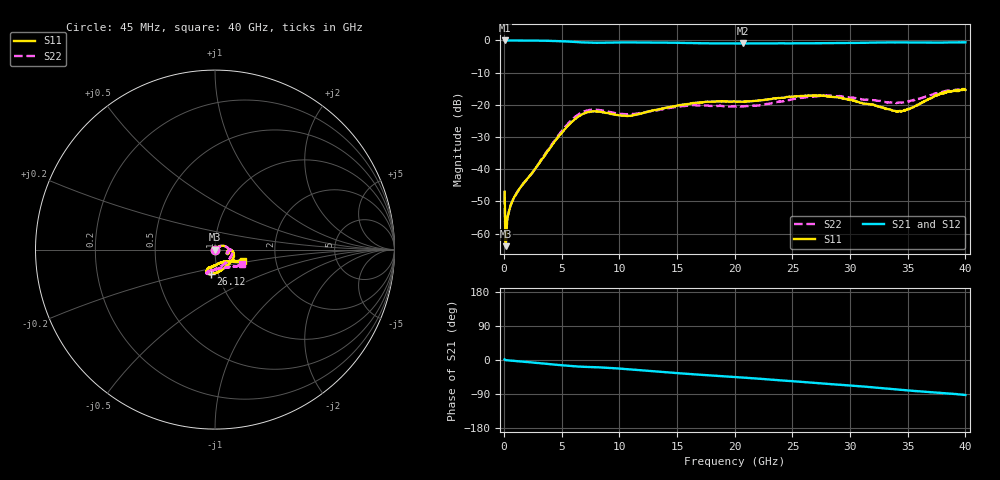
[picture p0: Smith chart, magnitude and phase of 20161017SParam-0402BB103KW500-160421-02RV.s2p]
! Board: 10mil Rogers 4350B, mounting pad dimensions: pad length=12.3 mils, pad width= 21 mils, pad gap=15.5 mils.
# GHZ S RI R 50
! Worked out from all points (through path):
!   801 points, 45 MHz to 40 GHz, reference 50 ohm
!   highest |S21| = 0.00 dB at 94.94 MHz (marker M1); lowest = -0.9 dB at 20.72 GHz (marker M2)
!   group delay of S21, straight-line fit = 6.22 ps
!   lowest |S11| = -63.9 dB at 144.9 MHz (marker M3), VSWR 1.00, Z = 50.1 - j0.0243 ohm
!   |S11| at or under -10 dB: start of sweep to end of sweep
!   |S22| runs from -63.6 to -15.1 dB; largest |S21 - S12| = 0.037
!   S11 on the Smith chart (normalised r, x): 45 MHz: 1.00, -0.01; 26.12 GHz: 0.92, -0.26; 40 GHz: 1.36, -0.18
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0.045  0.000548 -0.00445  0.988 0.031  1 -0.00352  0.00102 -0.0037
0.094944  0.000445 -0.00131  1 -0.00287  0.999 -0.00322  0.000416 -0.00116
0.144887  0.000589 -0.000243  0.999 -0.00615  0.999 -0.00622  0.00059 -0.000296
0.294719  0.00147 0.00101  0.998 -0.014  0.998 -0.014  0.00144 0.00102
0.544438  0.00207 0.00165  0.998 -0.025  0.998 -0.026  0.00212 0.00158
1.093819  0.00339 0.00258  0.996 -0.052  0.995 -0.051  0.00353 0.00244
4.290219  0.02 0.016  0.963 -0.202  0.962 -0.202  0.021 0.015
5.488869  0.041 0.022  0.93 -0.254  0.93 -0.254  0.045 0.02
6.737462  0.07 0.00889  0.889 -0.285  0.889 -0.285  0.076 0.00654
7.886169  0.078 -0.015  0.87 -0.299  0.87 -0.299  0.082 -0.017
10.78291  0.066 -0.015  0.85 -0.386  0.85 -0.386  0.069 -0.016
13.37998  0.085 -0.0016  0.799 -0.474  0.798 -0.474  0.083 -0.000114
16.32666  0.104 -0.02  0.723 -0.554  0.723 -0.554  0.098 -0.014
20.0225  0.08 -0.079  0.635 -0.634  0.635 -0.634  0.068 -0.066
20.72171  0.069 -0.088  0.618 -0.65  0.618 -0.65  0.057 -0.075
26.11564  -0.025 -0.137  0.473 -0.771  0.472 -0.772  -0.032 -0.127
26.71496  -0.033 -0.135  0.454 -0.782  0.454 -0.783  -0.039 -0.128
29.01237  -0.046 -0.121  0.384 -0.829  0.382 -0.827  -0.043 -0.129
33.35748  0.00721 -0.085  0.226 -0.905  0.224 -0.905  0.00945 -0.109
34.65602  0.041 -0.071  0.174 -0.916  0.174 -0.916  0.043 -0.101
37.80248  0.13 -0.065  0.055 -0.925  0.057 -0.923  0.126 -0.091
40  0.158 -0.065  -0.038 -0.936  -0.039 -0.94  0.153 -0.082
